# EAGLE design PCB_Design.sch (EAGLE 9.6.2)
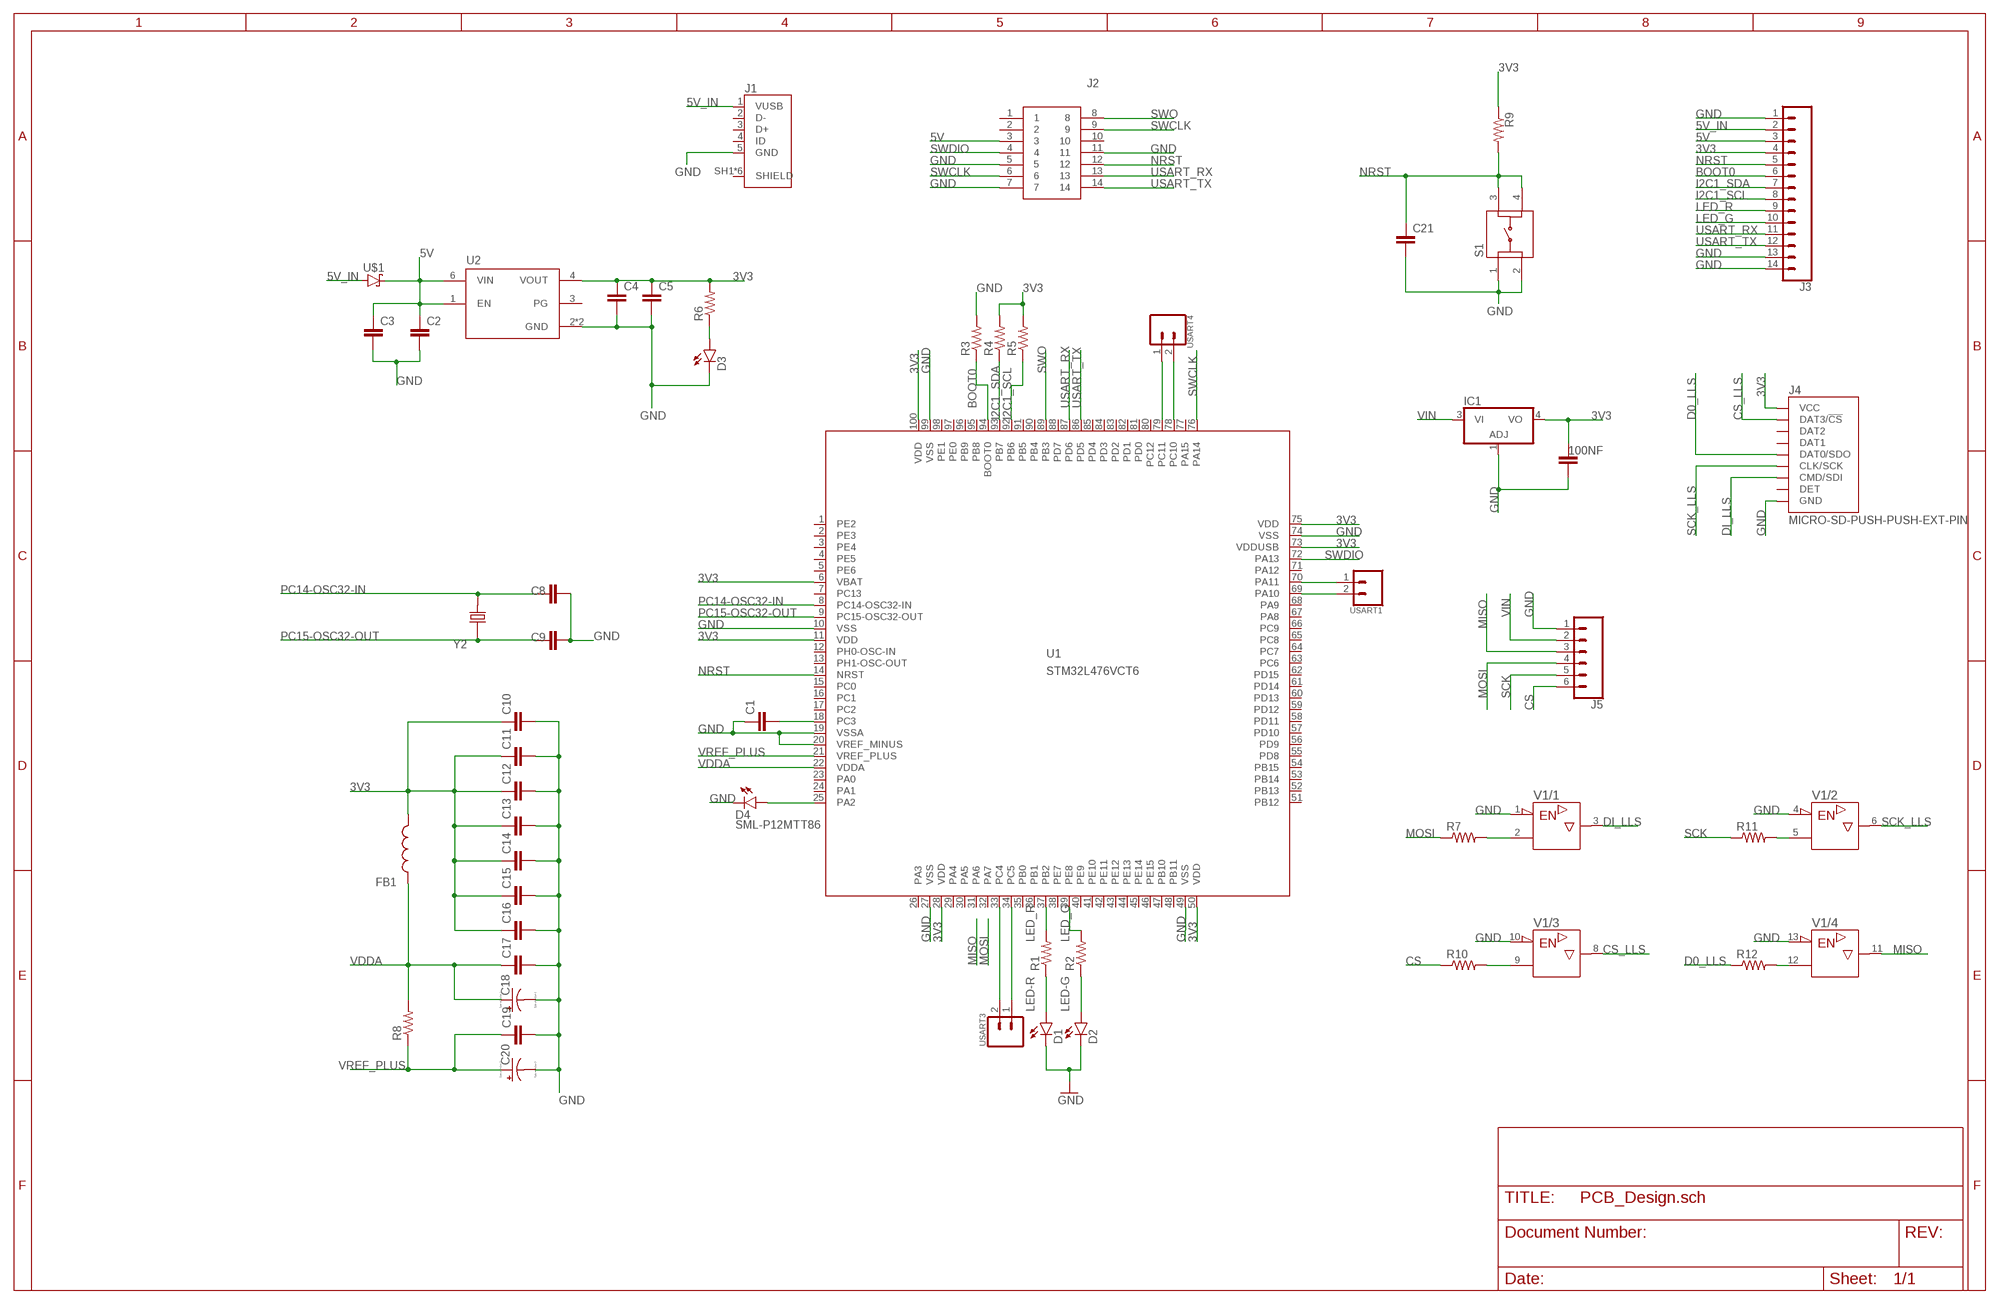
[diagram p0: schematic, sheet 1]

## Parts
100NF  C  (no package)
C1  CC0603KRX5R7BB105  [CAPC1608X90]
C2  CC0603KRX5R7BB105  [CAPC1608X90]
C3  CC0603KRX5R7BB105  [CAPC1608X90]
C4  CC0603KRX5R7BB105  [CAPC1608X90]
C5  CC0603KRX5R7BB105  [CAPC1608X90]
C8  CC0402CRNPO9BN4R7  [CAPC1005X55N]
C9  CC0402CRNPO9BN4R7  [CAPC1005X55N]
C10  CC0603KRX5R7BB105  [CAPC1608X90]
C11  CC0402KRX7R7BB104  [CAPC1005X55N]
C12  CC0402KRX7R7BB104  [CAPC1005X55N]
C13  CC0402KRX7R7BB104  [CAPC1005X55N]
C14  CC0402KRX7R7BB104  [CAPC1005X55N]
C15  CC0402KRX7R7BB104  [CAPC1005X55N]
C16  CC0402KRX7R7BB104  [CAPC1005X55N]
C17  CC0402KRX7R7BB104  [CAPC1005X55N]
C18  TAJA105K016RNJ  [CAPPM3216X180N]
C19  CC0402KRX7R7BB104  [CAPC1005X55N]
C20  TAJA105K016RNJ  [CAPPM3216X180N]
C21  CC0402KRX7R7BB104  [CAPC1005X55N]
D1  SML-P12MTT86  [LED_SML-P11UTT86R]
D2  SML-P12MTT86  [LED_SML-P11UTT86R]
D3  SML-P12VTT86  [LED_SML-P11UTT86R]
D4  SML-P12MTT86  [LED_SML-P11UTT86R]
FB1  BK1608HS601-T  [BEADC1608X95N]
IC1  317EMP  [SOT223]
J1  10118192-0001LF  [AMPHENOL_10118192-0001LF]
J2  FTSH-107-01-L-DV-K-A  [FTSH10701LDVKA]
J3  CONN_14  [1X14]
J4  MICRO-SD-PUSH-PUSH-EXT-PIN  [MICROSD-EXTERNALPIN]
J5  CONN_06LOCK  [1X06_LOCK]
R1  RC0402FR-071KL  [RESC1005X40N]
R2  RC0402FR-071KL  [RESC1005X40N]
R3  RC0402FR-071KL  [RESC1005X40N]
R4  RC0402FR-071KL  [RESC1005X40N]
R5  RC0402FR-071KL  [RESC1005X40N]
R6  RC0402FR-071KL  [RESC1005X40N]
R7  RC0402JR-070RL  [RESC1005X40]
R8  RC0402FR-071KL  [RESC1005X40N]
R9  RC0402FR-071KL  [RESC1005X40N]
R10  RC0402JR-070RL  [RESC1005X40]
R11  RC0402JR-070RL  [RESC1005X40]
R12  RC0402JR-070RL  [RESC1005X40]
S1  LL3301FF065QJ  [LL3301FF065QJ]
U1  STM32L476VCT6  [LQFP100_14X14]
U2  LD39050PU33R  [SON95P300X300X100-7N]
U$1  STPS1L30A  [DIOM5226X223N]
USART1  CONN_02LOCK  [1X02_LOCK]
USART3  CONN_02LOCK  [1X02_LOCK]
USART4  CONN_02LOCK  [1X02_LOCK]
V1  74125N  [DIL14]
Y2  ECS-.327-12.5-12QS-TR  [XTAL_ECS-.327-12.5-12QS-TR]

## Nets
3V3: 100NF.1 C4.1 C5.1 C10.1 C11.1 C12.1 C13.1 C14.1 C15.1 C16.1 FB1.2 IC1.4(VO) J3.4 J4.4(VCC) R4.2 R5.2 R6.2 R9.1 U1.6(VBAT) U1.11(VDD) U1.28(VDD) U1.50(VDD) U1.73(VDDUSB) U1.75(VDD) U1.100(VDD) U2.4(VOUT)
5V: C2.1 C3.1 J2.3 J3.3 U2.1(EN) U2.6(VIN) U$1.1(C)
5V_IN: J1.1(VUSB) J3.2 U$1.2(A)
BOOT0: J3.6 R3.1 U1.94(BOOT0)
CS: J5.6 R10.1
CS_LLS: J4.2(DAT3/!CS!) V1.8(/3:Y)
D0_LLS: J4.7(DAT0/SDO) R12.1
DI_LLS: J4.3(CMD/SDI) V1.3(/1:Y)
GND: 100NF.2 C1.1 C2.2 C3.2 C4.2 C5.2 C8.2 C9.2 C10.2 C11.2 C12.2 C13.2 C14.2 C15.2 C16.2 C17.2 C18.C(-) C19.2 C20.C(-) C21.2 D1.C D2.C D3.C D4.C IC1.1(ADJ) J1.5(GND) J2.5 J2.7 J2.11 J3.1 J3.13 J3.14 J4.6(GND) J4.10(GND) J4.11(GND) J4.12(GND) J4.13(GND) J5.1 R3.2 S1.1 S1.2 U1.10(VSS) U1.19(VSSA) U1.20(VREF_MINUS) U1.27(VSS) U1.49(VSS) U1.74(VSS) U1.99(VSS) U2.2(GND) U2.7(GND) V1.1(/1:!G) V1.4(/2:!G) V1.10(/3:!G) V1.13(/4:!G)
I2C1_SCL: J3.8 R5.1 U1.92(PB6)
I2C1_SDA: J3.7 R4.1 U1.93(PB7)
LED-G: D2.A R2.1
LED-R: D1.A R1.1
LED_G: J3.10 R2.2 U1.39(PE8)
LED_R: J3.9 R1.2 U1.37(PB2)
MISO: J5.3 V1.11(/4:Y)
MOSI: J5.4 R7.1
N$1: D4.A U1.25(PA2)
N$2: U1.33(PC4) USART3.2
N$3: U1.34(PC5) USART3.1
N$4: U1.78(PC10) USART4.2
N$5: U1.69(PA10) USART1.2
N$6: U1.79(PC11) USART4.1
N$7: U1.70(PA11) USART1.1
N$9: R7.2 V1.2(/1:A)
N$10: R10.2 V1.9(/3:A)
N$11: C1.2 U1.18(PC3)
N$13: R11.2 V1.5(/2:A)
N$14: D3.A R6.1
N$17: R12.2 V1.12(/4:A)
NRST: C21.1 J2.12 J3.5 R9.2 S1.3 S1.4 U1.14(NRST)
PC14-OSC32-IN: C8.1 U1.8(PC14-OSC32-IN) Y2.2
PC15-OSC32-OUT: C9.1 U1.9(PC15-OSC32-OUT) Y2.1
SCK: J5.5 R11.1
SCK_LLS: J4.5(CLK/SCK) V1.6(/2:Y)
SWCLK: J2.6 J2.9 U1.76(PA14)
SWDIO: J2.4 U1.72(PA13)
SWO: J2.8 U1.89(PB3)
USART_RX: J2.13 J3.11 U1.87(PD6)
USART_TX: J2.14 J3.12 U1.86(PD5)
VDDA: C17.1 C18.A(+) FB1.1 R8.2 U1.22(VDDA)
VIN: IC1.3(VI) J5.2
VREF_PLUS: C19.1 C20.A(+) R8.1 U1.21(VREF_PLUS)
Unconnected: J1.2(D-) J1.3(D+) J1.4(ID) J1.SH1(SHIELD) J1.SH2(SHIELD) J1.SH3(SHIELD) J1.SH4(SHIELD) J1.SH5(SHIELD) J1.SH6(SHIELD) J2.1 J2.2 J2.10 J4.1(DAT2) J4.8(DAT1) J4.9(DET) U1.1(PE2) U1.2(PE3) U1.3(PE4) U1.4(PE5) U1.5(PE6) U1.7(PC13) U1.12(PH0-OSC-IN) U1.13(PH1-OSC-OUT) U1.15(PC0) U1.16(PC1) U1.17(PC2) U1.23(PA0) U1.24(PA1) U1.26(PA3) U1.29(PA4) U1.30(PA5) U1.31(PA6) U1.32(PA7) U1.35(PB0) U1.36(PB1) U1.38(PE7) U1.40(PE9) U1.41(PE10) U1.42(PE11) U1.43(PE12) U1.44(PE13) U1.45(PE14) U1.46(PE15) U1.47(PB10) U1.48(PB11) U1.51(PB12) U1.52(PB13) U1.53(PB14) U1.54(PB15) U1.55(PD8) U1.56(PD9) U1.57(PD10) U1.58(PD11) U1.59(PD12) U1.60(PD13) U1.61(PD14) U1.62(PD15) U1.63(PC6) U1.64(PC7) U1.65(PC8) U1.66(PC9) U1.67(PA8) U1.68(PA9) U1.71(PA12) U1.77(PA15) U1.80(PC12) U1.81(PD0) U1.82(PD1) U1.83(PD2) U1.84(PD3) U1.85(PD4) U1.88(PD7) U1.90(PB4) U1.91(PB5) U1.95(PB8) U1.96(PB9) U1.97(PE0) U1.98(PE1) U2.3(PG)

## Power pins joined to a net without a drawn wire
+UB: V1.14(/+UB:+UB)
-UB: V1.7(/-UB:-UB)

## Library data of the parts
100NF = ngspice-simulation:C: CAPACITOR
C1-C5 C10 = ce-capstone:CC0603KRX5R7BB105: CAPACITOR CERAMIC, 1µF, 10V, X5R, 0603; Dielectric Characteristic:X5R; Capacitance:1µF; Capacitance Tolerance:± 10%; Voltage Rating:16V; Temperature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; DESCRIPTION: 1µF ±10% 16V Ceramic Capacitor X5R 0603 _1608 Metric_; DIGI-KEY_PART_NUMBER: 311-1444-1-ND; DIGI-KEY_PURCHASE_URL: https://www.digikey.com/product-detail/en/yageo/CC0603KRX5R7BB105/311-1444-1-ND/2833750?utm_source=snapeda&utm_medium=aggregator&utm_campaign=symbol; MF: Yageo; MP: CC0603KRX5R7BB105; PACKAGE: 0603 Yageo
C8 C9 = ce-capstone:CC0402CRNPO9BN4R7: 0402 4.7 pF 50 V ±0.25 pF Tolerance NP0 SMT Multilayer Ceramic Capacitor; DESCRIPTION: 4.7pF ±0.25pF 50V Ceramic Capacitor C0G, NP0 0402 _1005 Metric_; DIGI-KEY_PART_NUMBER: 311-1367-1-ND; DIGI-KEY_PURCHASE_URL: https://www.digikey.com/product-detail/en/yageo/CC0402CRNPO9BN4R7/311-1367-1-ND/2103151?utm_source=snapeda&utm_medium=aggregator&utm_campaign=symbol; MF: Yageo; MP: CC0402CRNPO9BN4R7; PACKAGE: 0402 Yageo
C11-C17 C19 C21 = ce-capstone:CC0402KRX7R7BB104: .1UF 16V 10% 0402; DESCRIPTION: 0.1µF ±10% 16V Ceramic Capacitor X7R 0402 _1005 Metric_; DIGI-KEY_PART_NUMBER: 311-1338-1-ND; DIGI-KEY_PURCHASE_URL: https://www.digikey.com/product-detail/en/yageo/CC0402KRX7R7BB104/311-1338-1-ND/2103122?utm_source=snapeda&utm_medium=aggregator&utm_campaign=symbol; MF: Yageo; MP: CC0402KRX7R7BB104; PACKAGE: 0402 Yageo
C18 C20 = ce-capstone:TAJA105K016RNJ: Capacitor tantalum TAJ 1206 1uF 16V AVX 1uF SMD Solid MnO2 Tantalum Electrolytic Capacitor, 16 V dc +/-10%, TAJ Series; ALLIED_NUMBER: 70474975; ALLIED_PRICE-STOCK: https://www.alliedelec.com/avx-taja105k016r/70474975/; DESCRIPTION: Capacitor tantalum TAJ 1206 1uF 16V AVX 1uF SMD Solid MnO2 Tantalum Electrolytic Capacitor, 16 V dc +/-10%, TAJ Series; HEIGHT: 1.8mm; MANUFACTURER_NAME: AVX; MANUFACTURER_PART_NUMBER: TAJA105K016RNJ; MOUSER_PART_NUMBER: 581-TAJA105K016RNJ; MOUSER_PRICE-STOCK: https://www.mouser.com/Search/Refine.aspx?Keyword=581-TAJA105K016R; RS_PART_NUMBER: 6992804P; RS_PRICE-STOCK: http://uk.rs-online.com/web/p/products/6992804P
D1 D2 D4 = ce-capstone:SML-P12MTT86: SML-P1 Series Red 0402 Clear 60 mcd 2 V Surface Mount PICOLED LED; AVAILABILITY: Unavailable; DESCRIPTION: Green 572nm LED Indication - Discrete 2V 0402 _1006 Metric_; MF: Rohm; MP: SML-P12MTT86; PACKAGE: 0402 Rohm; PRICE: None
D3 = ce-capstone:SML-P12VTT86: SML-P1 Series Red 0402 Clear 60 mcd 2 V Surface Mount PICOLED LED; AVAILABILITY: Unavailable; DESCRIPTION: Red 630nm LED Indication - Discrete 2V 0402 _1006 Metric_; MF: Rohm; MP: SML-P12VTT86; PACKAGE: 0402 Rohm; PRICE: None
FB1 = ce-capstone:BK1608HS601-T: Ferrite Chip Bead(Lead Free); DESCRIPTION: Ferrite Chip Bead(Lead Free); HEIGHT: 0.95mm; MANUFACTURER_NAME: Taiyo Yuden; MANUFACTURER_PART_NUMBER: BK1608HS601-T
IC1 = linear:*317: Positive VOLTAGE REGULATOR
J1 = ce-capstone:10118192-0001LF: Single Port 5 Contact Horizontal Right Angle Shielded Micro B USB 2.0 Connector; AVAILABILITY: Unavailable; DESCRIPTION: USB - micro B USB 2.0 Receptacle Connector 5 Position Surface Mount, Right Angle; MF: Amphenol ICC; MP: 10118192-0001LF; PACKAGE: None; PRICE: None
J2 = ce-capstone:FTSH-107-01-L-DV-K-A: Headers & Wire Housings .050" Micro Terminal Strip Source: Datasheet; DESCRIPTION: Headers & Wire Housings .050" Micro Terminal Strip; HEIGHT: 5.97mm; MANUFACTURER_NAME: SAMTEC; MANUFACTURER_PART_NUMBER: FTSH-107-01-L-DV-K-A; MOUSER_PART_NUMBER: 200-FTSH10701LDVKA; MOUSER_PRICE-STOCK: https://www.mouser.com/Search/Refine.aspx?Keyword=200-FTSH10701LDVKA
J3 = SparkFun-Connectors:CONN_14: Multi connection point. Often used as Generic Header-pin footprint for 0.1 inch spaced/style header connections On any of the 0.1 inch spaced packages, you can populate with these: Break Away Headers - Straight (PRT-00116) Break Away Male Headers - Right Angle (PRT-00553) Female Headers (PRT-00115)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
J4 = SparkFun-Connectors:MICRO-SD: microSD Socket for Transflash Various sockets for µSD. tDoc lines correctly indicate media card edge positions when inserting (unlocked, locked, depressed). NOTE: CD1 and CD2 are connected internally, and the default detect state of the socket is detect pin to ground. SparkFun Products: WAV Trigger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; PROD_ID: CONN-16110
J5 = SparkFun-Connectors:CONN_06: Multi connection point. Often used as Generic Header-pin footprint for 0.1 inch spaced/style header connections On any of the 0.1 inch spaced packages, you can populate with these: Break Away Headers - Straight (PRT-00116) Break Away Male Headers - Right Angle (PRT-00553) Female Headers (PRT-00115)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
R1-R6 R8 R9 = ce-capstone:RC0402FR-071KL: RES SMD 1k OHM 1% 1/16W 0402; DESCRIPTION: 510 Ohms ±1% 0.063W, 1/16W Chip Resistor 0402 _1005 Metric_ Moisture Resistant Thick Film; DIGI-KEY_PART_NUMBER: 311-510LRCT-ND; DIGI-KEY_PURCHASE_URL: https://www.digikey.com/product-detail/en/yageo/RC0402FR-07510RL/311-510LRCT-ND/729579?utm_source=snapeda&utm_medium=aggregator&utm_campaign=symbol; MF: Yageo; MP: RC0402FR-07510RL; PACKAGE: 1005 Panasonic Electronic Components
R7 R10-R12 = ce-capstone:RC0402JR-070RL: RC Series 0402 62.5 mW 0 Ohms 5% ±200 ppm/°C SMT Thick Film Chip Resistor; AVAILABILITY: Unavailable; DESCRIPTION: 0 Ohms Jumper 0.063W, 1/16W Chip Resistor 0402 _1005 Metric_ Moisture Resistant Thick Film; MF: Yageo; MP: RC0402JR-070RL; PACKAGE: 0402 Yageo; PRICE: None
S1 = ce-capstone:LL3301FF065QJ: Pushbutton Switches 50mA 12VDC F065 7.0mm J-Lead Source: Datasheet; DESCRIPTION: Pushbutton Switches 50mA 12VDC F065 7.0mm J-Lead; HEIGHT: 7.3mm; MANUFACTURER_NAME: E-Switch; MANUFACTURER_PART_NUMBER: LL3301FF065QJ; MOUSER_PART_NUMBER: 612-LL3301FF065QJ; MOUSER_PRICE-STOCK: https://www.mouser.com/Search/Refine.aspx?Keyword=612-LL3301FF065QJ
U1 = ce-capstone:STM32L476V*: STM32L476VX LQFP100 Datasheet STM32L476XX; FARNELL: 2518171; FLASH: 256kB; SRAM: 128kB
U2 = ce-capstone:LD39050PU33R: LD39050 Series 500 mA 3.3 V Fixed Low Noise LDO Voltage Regulator - DFN-6; AVAILABILITY: Unavailable; DESCRIPTION: Linear Voltage Regulator IC 1 Output 500mA 6-DFN _3x3_; MF: STMicroelectronics; MP: LD39050PU33R; PACKAGE: DFN-6 STMicroelectronics; PRICE: None
U$1 = ce-capstone:STPS1L30A
USART1 USART3 USART4 = SparkFun-Connectors:CONN_02: Multi connection point. Often used as Generic Header-pin footprint for 0.1 inch spaced/style header connections
V1 = 74ttl-din:74*125: Quad bus BUFFER, 3-state
Y2 = ce-capstone:ECS-.327-12.5-12QS-TR: SMD CRYSTAL 32.768 KHz; AVAILABILITY: Unavailable; DESCRIPTION: 32.768kHz ±20ppm Crystal 12.5pF 90 kOhms 2-SMD, No Lead; MF: ECS Inc.; MP: ECS-.327-12.5-12QS-TR; PACKAGE: SMD-2 ECS International; PRICE: None

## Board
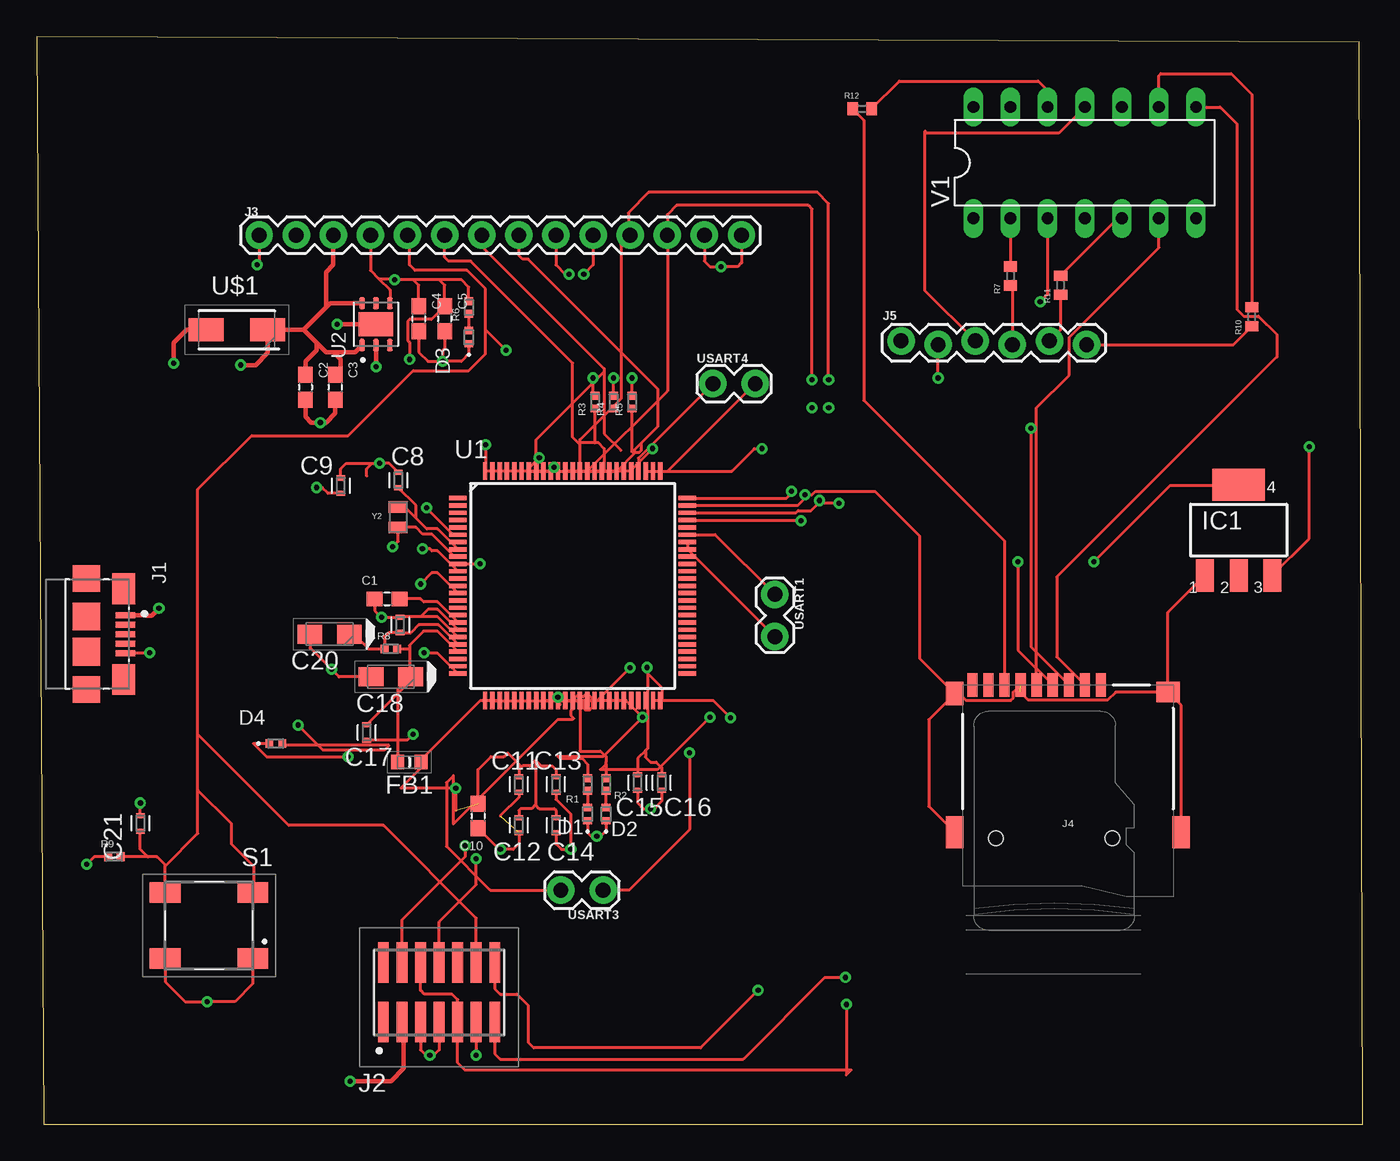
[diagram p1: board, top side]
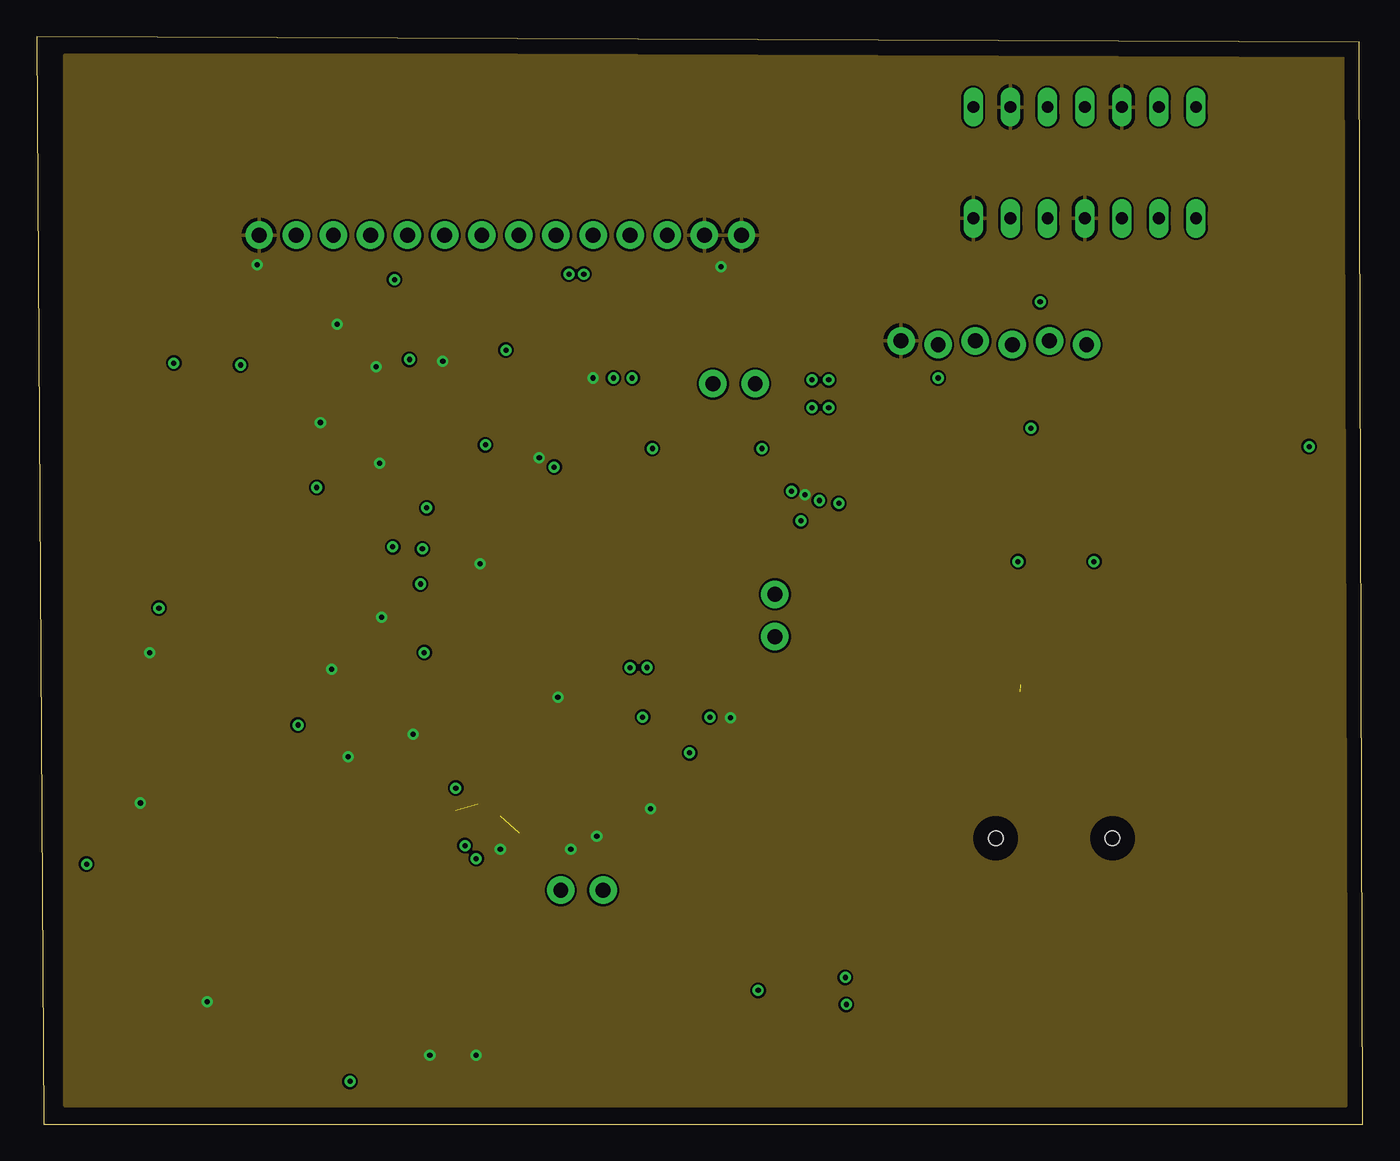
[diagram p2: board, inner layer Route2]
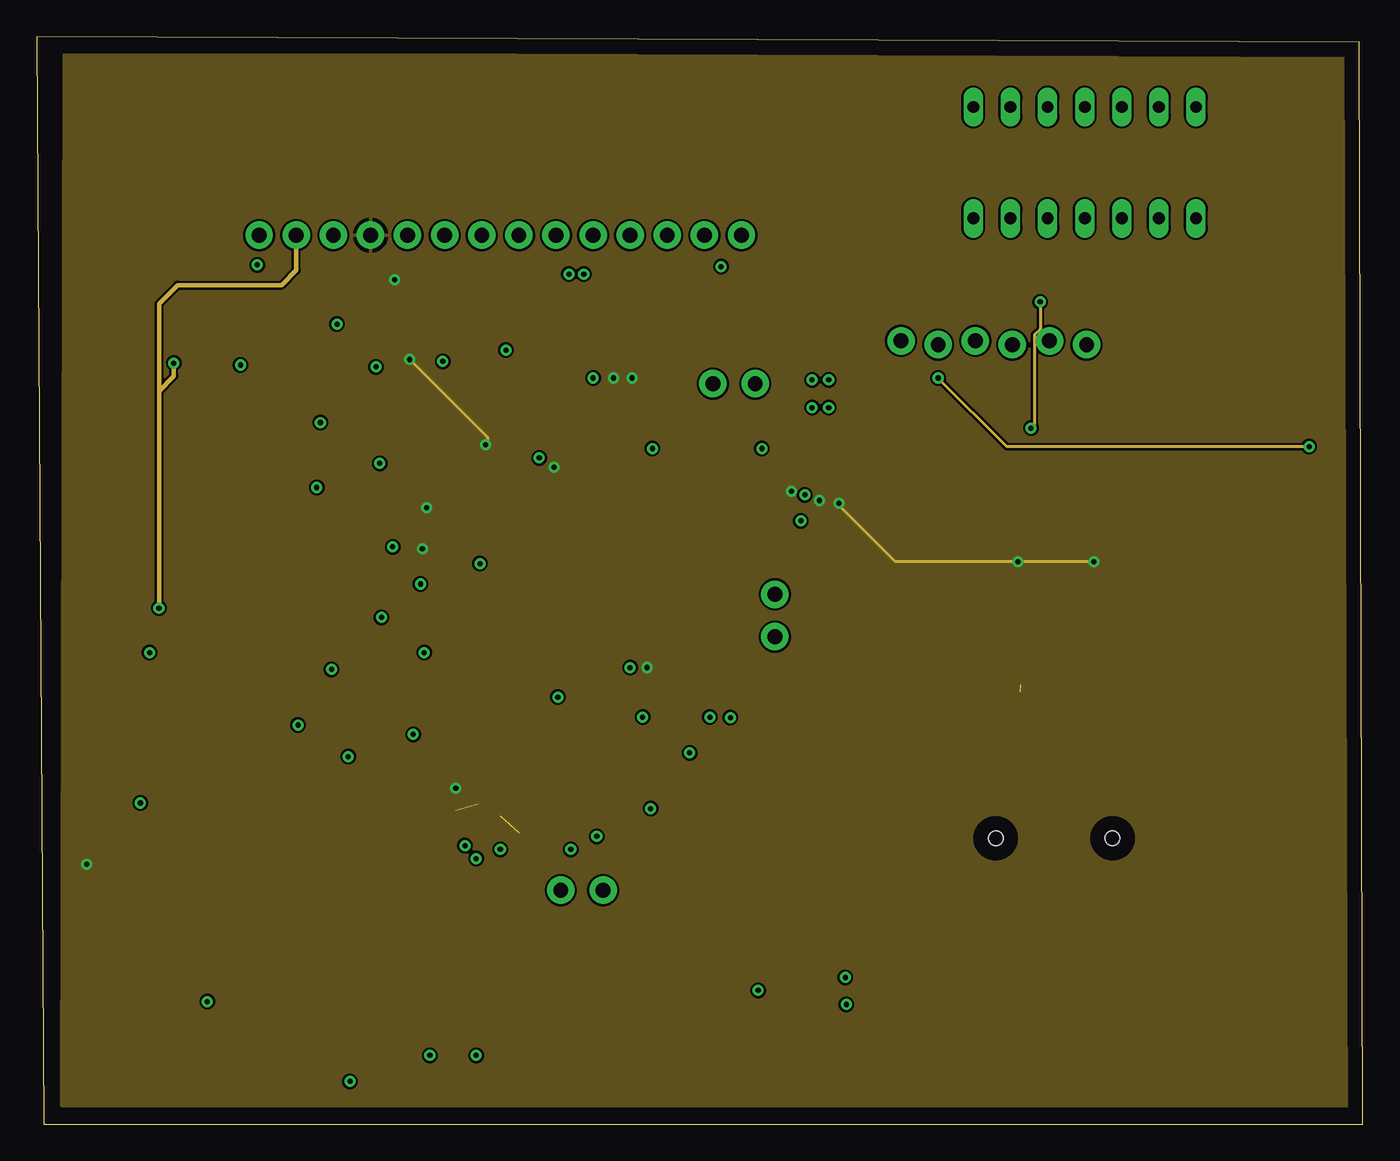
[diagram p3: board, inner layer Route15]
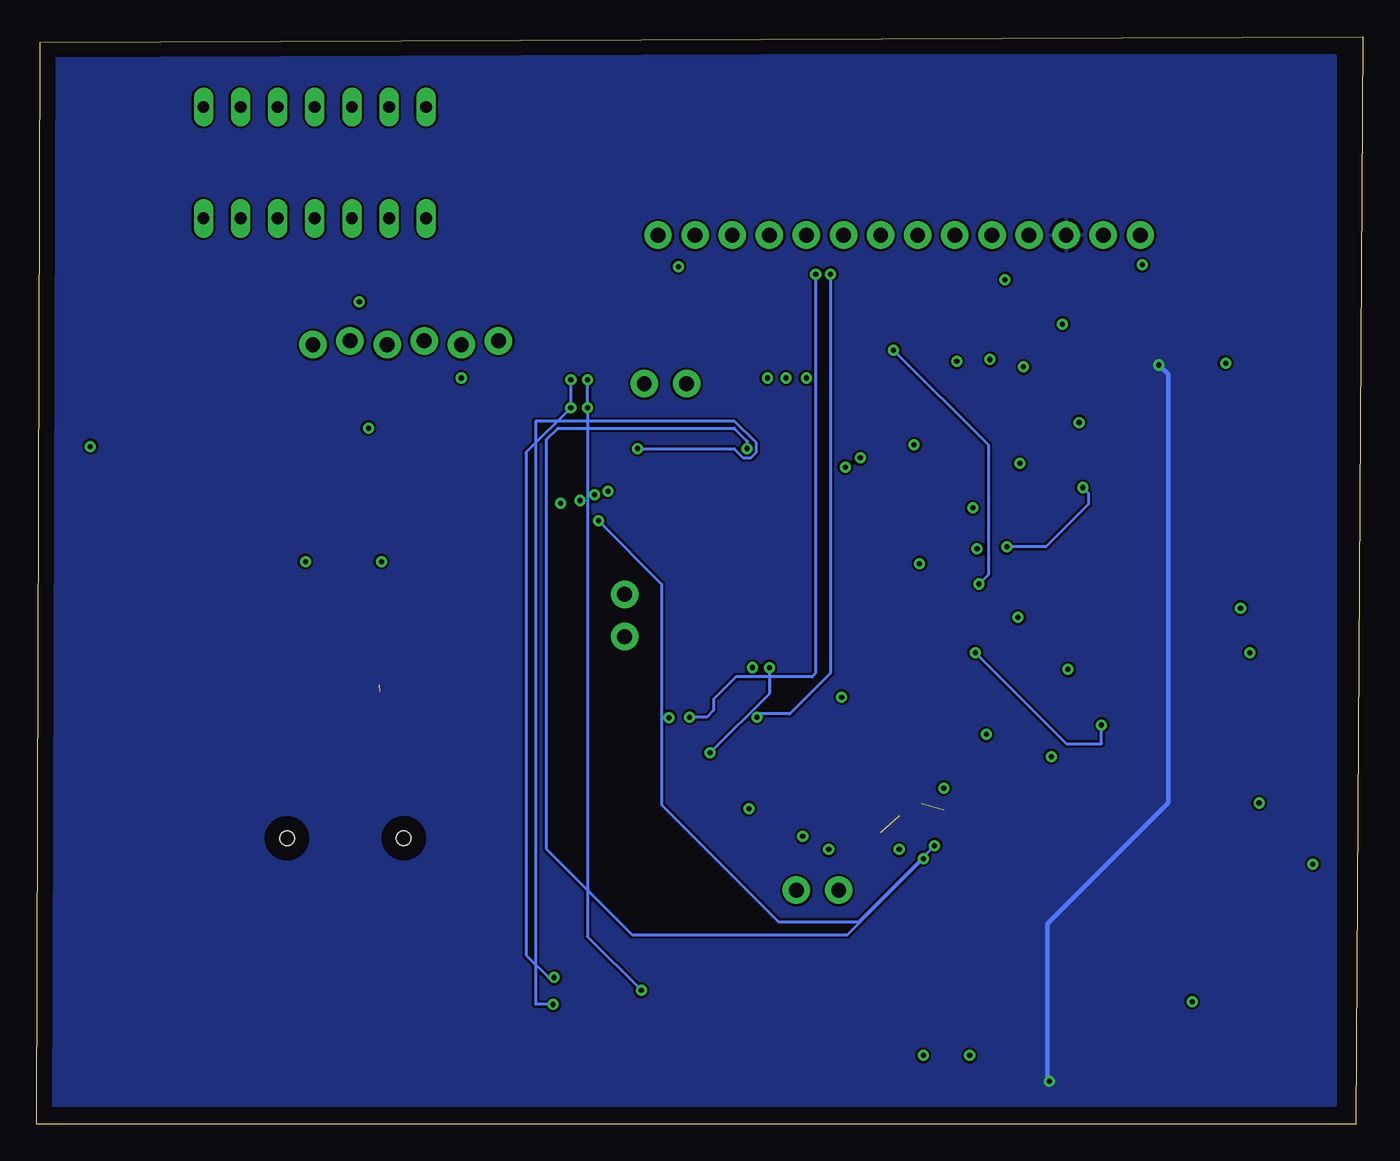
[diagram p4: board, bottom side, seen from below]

Size 90.81 x 74.42 mm. Coordinates in mm from the lower left corner, seen from the top.
Outline: 0.51,0 90.81,0 90.55,74.04 0,74.42 0.51,0
Copper layers (1+2*15+16): Top 0.035mm / dielectric 1.5mm / Route2 0.035mm / dielectric 0.15mm / Route15 0.035mm / dielectric 0.2mm / Bottom 0.035mm
Design rules "default *": minimum track width 8mil, minimum drill 0.35mm, track to track 6mil, track to pad 6mil, pad to pad 6mil, via to via 6mil, smd to smd 6mil, copper to edge 40mil, drill to drill 6mil, minimum pad ring 10mil, minimum via ring 8mil, stop-mask expansion 4mil, vias tented up to drill 0mil, thermal gap 10mil

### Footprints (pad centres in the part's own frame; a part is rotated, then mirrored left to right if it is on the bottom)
CAPC1608X90 = smd 1.1 x 1: 1 -0.85,0; 2 0.85,0
CAPC1005X55N = smd 0.35 x 0.6: 1 -0.525,0; 2 0.525,0
CAPPM3216X180N = smd 1.7 x 1.3: A -1.35,0; C 1.35,0
LED_SML-P11UTT86R = smd 0.5 x 0.6: A 0.45,0; C -0.45,0
BEADC1608X95N = smd 0.9 x 1: 1 -0.8,0; 2 0.8,0
SOT223 = smd 1.219 x 2.235: 1 -2.311,-3.099; 2 0,-3.099; 3 2.311,-3.099 | smd 3.6 x 2.2: 4 0,3.099
AMPHENOL_10118192-0001LF = smd 0.4 x 1.35: 1 -1.3,0; 2 -0.65,0; 3 0,0; 4 0.65,0; 5 1.3,0 | smd 2.1 x 1.6: SH1 -3.1,-0.125; SH2 3.1,-0.125 | smd 1.8 x 1.9: SH3 -3.8,-2.675; SH6 3.8,-2.675 | smd 1.9 x 1.9: SH4 -1.2,-2.675; SH5 1.2,-2.675
FTSH10701LDVKA = smd 0.74 x 2.79: 1 -3.81,-2.035; 2 -3.81,2.035; 3 -2.54,-2.035; 4 -2.54,2.035; 5 -1.27,-2.035; 6 -1.27,2.035; 7 0,-2.035; 8 0,2.035; 9 1.27,-2.035; 10 1.27,2.035; 11 2.54,-2.035; 12 2.54,2.035; 13 3.81,-2.035; 14 3.81,2.035
1X14 = drill 1.016 pad 1.88: 1 0,0; 2 2.54,0; 3 5.08,0; 4 7.62,0; 5 10.16,0; 6 12.7,0; 7 15.24,0; 8 17.78,0; 9 20.32,0; 10 22.86,0; 11 25.4,0; 12 27.94,0; 13 30.48,0; 14 33.02,0
MICROSD-EXTERNALPIN = smd 0.7 x 1.6: 1 2.25,10.5; 2 1.15,10.5; 3 0.05,10.5; 4 -1.05,10.5; 5 -2.15,10.5; 6 -3.25,10.5; 7 -4.35,10.5; 8 -5.45,10.5; 9 -6.55,10.5 | smd 1.2 x 1.6: 10 -7.75,9.9 | smd 1.2 x 2.2: 11 -7.75,0.4; 12 7.75,0.4 | smd 1.6 x 1.4: 13 6.85,10 | hole 1: 3.05,0; -4.95,0
1X06_LOCK = drill 1.016 pad 1.88: 1 0,0; 2 2.54,-0.254; 3 5.08,0; 4 7.62,-0.254; 5 10.16,0; 6 12.7,-0.254
RESC1005X40N = smd 0.54 x 0.6: 1 -0.432,0; 2 0.432,0
RESC1005X40 = smd 0.7 x 0.9: 1 -0.65,0; 2 0.65,0
LL3301FF065QJ = smd 2.1 x 1.4: 1 -3,2.25; 2 3,2.25; 3 -3,-2.25; 4 3,-2.25
LQFP100_14X14 = smd 1.2 x 0.3: 1 -7.85,6; 2 -7.85,5.5; 3 -7.85,5; 4 -7.85,4.5; 5 -7.85,4; 6 -7.85,3.5; 7 -7.85,3; 8 -7.85,2.5; 9 -7.85,2; 10 -7.85,1.5; 11 -7.85,1; 12 -7.85,0.5; 13 -7.85,0; 14 -7.85,-0.5; 15 -7.85,-1; 16 -7.85,-1.5; 17 -7.85,-2; 18 -7.85,-2.5; 19 -7.85,-3; 20 -7.85,-3.5; 21 -7.85,-4; 22 -7.85,-4.5; 23 -7.85,-5; 24 -7.85,-5.5; 25 -7.85,-6; 51 7.85,-6; 52 7.85,-5.5; 53 7.85,-5; 54 7.85,-4.5; 55 7.85,-4; 56 7.85,-3.5; 57 7.85,-3; 58 7.85,-2.5; 59 7.85,-2; 60 7.85,-1.5; 61 7.85,-1; 62 7.85,-0.5; 63 7.85,0; 64 7.85,0.5; 65 7.85,1; 66 7.85,1.5; 67 7.85,2; 68 7.85,2.5; 69 7.85,3; 70 7.85,3.5; 71 7.85,4; 72 7.85,4.5; 73 7.85,5; 74 7.85,5.5; 75 7.85,6 | smd 0.3 x 1.2: 26 -6,-7.85; 27 -5.5,-7.85; 28 -5,-7.85; 29 -4.5,-7.85; 30 -4,-7.85; 31 -3.5,-7.85; 32 -3,-7.85; 33 -2.5,-7.85; 34 -2,-7.85; 35 -1.5,-7.85; 36 -1,-7.85; 37 -0.5,-7.85; 38 0,-7.85; 39 0.5,-7.85; 40 1,-7.85; 41 1.5,-7.85; 42 2,-7.85; 43 2.5,-7.85; 44 3,-7.85; 45 3.5,-7.85; 46 4,-7.85; 47 4.5,-7.85; 48 5,-7.85; 49 5.5,-7.85; 50 6,-7.85; 76 6,7.85; 77 5.5,7.85; 78 5,7.85; 79 4.5,7.85; 80 4,7.85; 81 3.5,7.85; 82 3,7.85; 83 2.5,7.85; 84 2,7.85; 85 1.5,7.85; 86 1,7.85; 87 0.5,7.85; 88 0,7.85; 89 -0.5,7.85; 90 -1,7.85; 91 -1.5,7.85; 92 -2,7.85; 93 -2.5,7.85; 94 -3,7.85; 95 -3.5,7.85; 96 -4,7.85; 97 -4.5,7.85; 98 -5,7.85; 99 -5.5,7.85; 100 -6,7.85
SON95P300X300X100-7N = smd 0.84 x 0.4: 1 -1.435,0.95; 2 -1.435,0; 3 -1.435,-0.95; 4 1.435,-0.95; 5 1.435,0; 6 1.435,0.95 | smd 1.625 x 2.365: 7 0,0
DIOM5226X223N = smd 2.4 x 1.55: 1 -2.1,0; 2 2.1,0
1X02_LOCK = drill 1.016 pad 1.88: 1 -0.178,0; 2 2.718,0
DIL14 = drill 0.813 long: 1 -7.62,-3.81; 2 -5.08,-3.81; 3 -2.54,-3.81; 4 0,-3.81; 5 2.54,-3.81; 6 5.08,-3.81; 7 7.62,-3.81; 8 7.62,3.81; 9 5.08,3.81; 10 2.54,3.81; 11 0,3.81; 12 -2.54,3.81; 13 -5.08,3.81; 14 -7.62,3.81
XTAL_ECS-.327-12.5-12QS-TR = smd 0.8 x 1.3: 1 -0.7,0; 2 0.7,0

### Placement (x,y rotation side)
C1  24,35.94 0 top
C2  18.42,50.42 270 top
C3  20.45,50.42 270 top
C4  26.16,55.12 270 top
C5  27.94,55.12 270 top
C8  24.77,44.07 90 top
C9  20.83,43.69 90 top
C10  30.23,21.08 270 top
C11  33.02,23.24 270 top
C12  33.02,20.45 270 top
C13  35.56,23.24 270 top
C14  35.56,20.45 270 top
C15  41.15,23.37 270 top
C16  42.8,23.37 270 top
C17  22.61,26.8 270 top
C18  24.26,30.61 180 top
C19  24.89,34.16 90 top
C20  20.07,33.53 180 top
C21  7.11,20.57 90 top
D1  37.72,21.21 90 top
D2  38.99,21.21 90 top
D3  29.59,53.85 90 top
D4  16.38,26.04 0 top
FB1  25.53,24.77 0 top
IC1  82.3,40.64 0 top
J1  6.1,33.53 270 top
J2  27.56,9.02 0 top
J3  15.24,60.83 0 top
J4  70.61,19.56 0 top
J5  59.18,53.59 0 top
R1  37.72,23.24 90 top
R2  38.99,23.24 90 top
R3  38.23,49.4 90 top
R4  39.5,49.4 90 top
R5  40.77,49.4 90 top
R6  29.59,55.88 90 top
R7  66.68,58.04 90 top
R8  24.26,32.51 0 top
R9  5.33,18.29 0 top
R10  83.19,55.24 90 top
R11  70.1,57.4 90 top
R12  56.52,69.47 0 top
S1  11.81,13.59 180 top
U1  36.7,36.83 0 top
U2  23.24,54.74 90 top
U$1  13.72,54.36 180 top
USART1  50.55,36.07 270 top
USART3  38.61,16 180 top
USART4  46.48,50.67 0 top
V1  71.76,65.79 0 top
Y2  24.77,41.53 90 top

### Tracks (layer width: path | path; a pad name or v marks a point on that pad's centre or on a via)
3V3  (via drill 0.35)  (1 unrouted)
  Top 0.203: U1.28 30.38,28.98 26.33,24.93 FB1.2 26.33,24.38 24.93,22.99 v28.7,22.99 28.7,21.46 | U1.50 42.83,29.11 42.83,29.84 41.81,30.86 | 41.81,30.86 41.81,25.68 41.69,25.56 | 41.69,25.56 41.15,25.02 C15.1 | 41.69,25.56 41.69,25.11 42.04,24.77 42.42,24.77 42.8,24.38 C16.1 | 34.16,24.89 33.78,24.51 33.27,24.51 33.02,24.26 C11.1 33.02,24.64 32.26,25.4 32,25.15 31.12,25.15 30.23,24.26 C10.1 | 34.16,24.89 34.54,24.51 35.31,24.51 35.56,24.26 C13.1 | 34.16,24.89 34.16,21.84 | 34.16,21.84 33.91,21.59 33.15,21.59 33.02,21.46 C12.1 | 34.16,21.84 34.42,21.59 35.43,21.59 35.56,21.46 C14.1 | R4.2 v39.5,51.05 | R5.2 v40.77,51.05 | v41.78,31.24 41.78,30.89 41.81,30.86 | J3.4 22.86,58.42 23.43,57.85 | U2.4 24.19,57.09 23.43,57.85 | 23.43,57.85 24.45,57.85 v24.51,57.78 25.78,57.78 | C4.1 26.16,57.4 25.78,57.78 | 27.56,57.78 27.94,57.4 C5.1 27.04,55.07 25.56,55.07 25.41,54.92 25.41,53.61 25.53,53.49 v25.53,52.32 | 27.56,57.78 25.78,57.78 | R6.2 29.59,57.28 29.08,57.78 27.56,57.78 | R9.1 3.94,18.29 v3.43,17.78 | U1.75 51.34,42.83 51.69,43.18 v51.69,43.31 | U1.73 51.98,41.83 52.13,41.97 53.02,41.97 53.59,42.55 v53.59,42.67 53.78,42.48 v54.93,42.48 | U1.6 28.5,40.33 26.71,42.13 v26.71,42.16 | U1.11 27.46,39.23 27.07,39.23 26.94,39.36 v26.42,39.36 | v35.43,44.96 35.16,44.68 30.8,44.68 | 30.8,44.68 U1.100 | IC1.4 82.25,43.69 77.6,43.69 v72.39,38.48 | v67.18,38.48 67.18,32.44 J4.4 | v30.73,46.48 30.73,44.81 30.8,44.74 30.8,44.68
  Route15 0.203: v72.39,38.48 v67.18,38.48 58.8,38.48 54.86,42.42 v54.93,42.48 | v25.53,52.32 30.86,46.99 30.86,46.61 v30.73,46.48
  pour Route15: 1.7,1.27 89.79,1.27 89.79,73.15 1.86,73.15
5V  (via drill 0.35)
  Top 0.305: 18.29,54.36 U$1.1 15.82,52.77 14.99,51.94 v13.97,51.94 | J3.3 20.32,58.8 19.81,58.29 19.81,55.88 | 18.29,54.36 19.81,55.88 | 19.81,55.88 20.1,56.17 U2.6 | 18.29,54.36 19.18,53.47 | 19.18,53.47 19.18,52.96 18.42,52.2 C2.1 | 19.18,53.47 19.81,52.83 20.32,52.83 | U2.1 21.82,52.83 20.32,52.83 | 20.32,52.83 20.83,52.32 20.83,51.65 C3.1 | v21.46,2.92 24.26,2.92 25.15,3.81 25.15,6.86 J2.3
  Bottom 0.305: v13.97,51.94 13.33,51.31 13.33,21.97 21.59,13.72 21.59,3.05 v21.46,2.92
  pour Bottom: 1.91,73.15 1.91,1.27 89.79,1.27 89.79,73.15
5V_IN  (via drill 0.35)
  Top 0.305: J1.1 7.46,34.83 7.49,34.8 7.87,34.8 v8.38,35.31 | v9.4,52.07 9.4,53.47 10.29,54.36 U$1.2
  Route15 0.305: v8.38,35.31 8.38,50.16 | 8.38,50.16 8.38,53.21 8.38,56.13 9.65,57.4 16.76,57.4 17.78,58.42 J3.2 | 8.38,50.16 9.4,51.18 v9.4,52.07
BOOT0
  Top 0.203: U1.94 38.86,44.68 38.86,46.23 38.48,46.61 38.23,46.61 | 38.23,46.61 R3.1 | 38.23,46.61 37.08,46.61 36.7,46.99 36.7,52.07 29.72,59.05 28.19,59.05 27.94,59.31 J3.6
CS
  Top 0.203: J5.6 81.93,53.34 R10.1
CS_LLS
  Top 0.203: V1.8 81.03,69.6 82.17,68.45 82.17,55.75 82.63,55.29 83.65,55.29 84.91,54.03 84.91,52.5 69.84,37.44 69.84,31.98 J4.2
D0_LLS
  Top 0.203: R12.1 56.64,68.69 56.64,49.53 66.26,39.91 J4.7
DI_LLS  (via drill 0.35)
  Top 0.203: V1.3 69.22,56.77 v68.71,56.26 | v68.07,47.62 68.07,32.65 J4.3
  Route15 0.203: v68.71,56.26 68.71,54.4 68.33,54.02 68.33,47.88 v68.07,47.62
GND  (via drill 0.35)  (2 unrouted)
  Top 0.203: J1.5 6.13,32.26 v7.75,32.26 | U1.20 27.46,34.73 26.29,34.73 | 26.29,34.73 24.93,34.73 C19.2 24.89,34.67 v23.62,34.67 23.15,35.14 C1.1 | U1.19 27.46,35.23 26.79,35.23 26.29,34.73 | C20.C 18.72,32.59 v20.19,31.11 20.7,30.61 C18.C | v25.78,26.67 25.38,26.27 C17.2 | C13.2 35.56,22.23 36.58,21.21 v36.58,18.8 35.94,18.8 35.56,19.18 C14.2 | C11.2 33.02,22.35 31.75,21.08 | C15.2 41.15,21.97 41.53,21.59 v42.04,21.59 42.29,21.59 42.8,22.1 C16.2 | v47.5,27.81 46.33,28.98 U1.49 | C10.2 31.66,18.8 v31.75,18.8 32.64,18.8 33.02,19.18 C12.2 | D1.C 37.72,19.94 37.97,19.69 v38.35,19.69 38.61,19.69 38.99,20.07 D2.C | C8.2 24.15,45.21 v23.5,45.21 22.99,45.21 | 22.61,44.34 22.61,44.83 22.99,45.21 | C9.2 20.83,44.83 21.21,45.21 22.99,45.21 | D3.C 29.59,52.7 29.08,52.2 v27.81,52.2 | C5.2 27.94,53.09 27.81,52.96 v27.81,52.2 | C4.2 26.16,52.83 26.8,52.2 v27.81,52.2 | S1.2 8.81,9.73 10.16,8.38 v11.68,8.38 13.59,8.38 14.81,9.6 S1.1 | C21.2 v7.11,21.97 | J2.5 26.29,5.08 26.67,4.7 v26.92,4.7 27.18,4.7 27.56,5.08 J2.7 | J2.11 v30.1,4.7 | J3.13 45.72,59.05 46.1,58.67 v46.86,58.67 48.01,58.67 48.26,58.93 J3.14 | U1.74 52.11,42.33 52.6,42.82 v52.6,43.05 53.08,43.05 53.33,43.3 57.41,43.3 60.45,40.26 60.45,31.87 J4.10 | v15.11,58.8 15.24,58.93 J3.1 | U1.10 30.35,38.33 v30.35,38.35 | v34.42,45.59 33.5,44.68 U1.99 | U1.27 35.56,28.98 35.84,28.7 35.81,28.7 35.69,28.83 v35.69,29.21 | R3.2 38.1,49.96 v38.1,51.05 | D4.C 14.86,26.04 15.75,25.15 v21.34,25.15 | J4.12 78.36,28.66 J4.13 | J4.13 77.46,35.02 IC1.1 | J4.10 61.09,27.68 61.09,21.73 J4.11 | J4.13 73.87,29.56 73.32,29 67.9,29 67.31,29.59 | 66.72,29 | 66.72,29 66.87,29.15 66.87,29.56 J4.6
  Top 0.203: J4.10 63.15,29.46 63.61,29 66.72,29
  Top 0.305: C2.2 18.42,48.39 18.8,48.01 v19.43,48.01 19.81,48.01 20.45,48.64 C3.2 | U2.2 v23.24,51.82 | U2.7 v20.57,54.74
  pour Route2: 1.91,73.15 1.91,1.27 89.66,1.27 89.66,73.15
I2C1_SCL
  Top 0.203: U1.92 39.73,44.68 41.02,45.97 41.27,45.97 41.4,46.1 41.4,46.61 | R5.1 40.77,45.97 41.4,46.61 | 41.4,46.61 42.54,47.75 42.54,50.29 33.66,59.18 33.27,59.18 33.02,59.44 J3.8
I2C1_SDA
  Top 0.203: 38.86,51.5 34.2,46.84 U1.93 | 38.86,51.5 38.86,51.69 30.48,60.07 J3.7 | 38.86,51.5 38.86,47.24 40,46.1
LED-G
  Top 0.203: D2.A R2.1
LED-R
  Top 0.203: R1.1 D1.A
LED_G  (via drill 0.35)
  Top 0.203: U1.39 37.2,25.53 38.61,25.53 38.99,25.15 38.99,24.77 38.99,24.64 | 38.99,24.64 R2.2 | J3.10 38.1,58.8 v37.46,58.17 | v46.1,27.85 42.51,24.26 38.61,24.26 38.99,24.64
  Bottom 0.203: v37.46,58.17 37.46,30.86 37.72,30.61 42.93,30.61 44.45,29.08 44.45,28.32 44.92,27.85 v46.1,27.85
LED_R  (via drill 0.35)
  Top 0.203: U1.37 40.37,28.98 v41.5,27.85 38.79,25.14 35.7,25.14 35.81,25.02 37.34,25.02 37.72,24.64 R1.2 | J3.9 35.56,58.8 36.2,58.17 v36.45,58.17
  Bottom 0.203: v36.45,58.17 36.45,30.86 39.24,28.07 41.28,28.07 v41.5,27.85
MISO
  Top 0.203: J5.3 60.83,57.02 60.83,67.82 | 60.83,67.82 60.83,67.94 | V1.11 69.98,67.82 60.83,67.82
MOSI
  Top 0.203: R7.1 66.8,57.26 J5.4
N$1  (via drill 0.35)
  Top 0.203: U1.25 27.46,32.23 26.57,32.23 v26.54,32.26 | v17.91,27.3 19.62,25.6 23.82,25.6 24.13,25.91 16.96,25.91 D4.A
  Bottom 0.203: v26.54,32.26 20.32,26.04 17.91,26.04 v17.91,27.3
N$2
  Top 0.203: U1.33 37.43,28.98 37.43,28.49 37.57,28.35 37.87,28.35 38.07,28.55 38.07,28.85 38.03,28.9 38.03,29.13 37.82,29.34 37.52,29.34 37.42,29.23 37.32,29.34 37.02,29.34 36.72,29.03 36.72,28.42 36.57,28.27 36.57,27.98 36.78,27.77 36.69,27.68 35.68,27.68 28.54,20.54 28.54,23.84 28.07,23.37 28.07,19 31.06,16 USART3.2
N$3  (via drill 0.35)
  Top 0.203: v40.64,31.24 38.38,28.98 U1.34 | v44.7,25.4 44.7,20.14 40.56,16 USART3.1
  Bottom 0.203: v40.64,31.24 40.64,29.46 v44.7,25.4
N$4
  Top 0.203: U1.78 43.21,44.68 USART4.2
N$5
  Top 0.203: U1.69 44.55,39.34 USART1.2
N$6
  Top 0.203: USART4.1 41.2,45.57 U1.79
N$7
  Top 0.203: U1.70 46.46,40.33 USART1.1
N$9
  Top 0.203: V1.2 R7.2
N$10
  Top 0.203: V1.9 76.84,71.75 76.96,71.88 81.79,71.88 83.19,70.49 R10.2
N$11
  Top 0.203: U1.18 27.46,35.73 26.5,35.73 26.29,35.94 C1.2
N$13
  Top 0.203: R11.2 74.03,61.98 V1.5
N$14
  Top 0.203: R6.1 D3.A
N$17
  Top 0.203: R12.2 59.07,71.37 68.58,71.37 69.22,70.74 V1.12
NRST  (via drill 0.35)
  Top 0.203: S1.4 8.81,17.65 | 8.81,17.65 8.81,17.73 8.25,18.29 7.62,18.29 | 7.62,18.29 R9.2 | 7.62,18.29 7.11,18.8 C21.1 | S1.3 14.86,15.89 14.86,17.65 13.33,19.18 13.33,20.57 11.05,22.86 | 8.81,17.65 11.05,19.89 11.05,22.86 | 11.05,22.86 11.05,26.67 | 11.05,26.67 11.05,43.43 14.73,47.12 21.34,47.12 25.78,51.56 29.59,51.56 30.73,52.7 30.73,54.36 | 30.73,54.36 30.73,57.15 29.46,58.42 25.91,58.42 25.53,58.8 25.53,60.71 J3.5 | J2.12 30.1,14.1 23.75,20.45 17.27,20.45 11.05,26.67 | U1.14 27.46,37.73 27.06,37.73 v26.29,36.96 | v32.13,52.96 30.73,54.36
  Bottom 0.203: v26.29,36.96 25.65,37.59 25.65,46.48 v32.13,52.96
PC14-OSC32-IN
  Top 0.203: U1.8 27.46,40.73 26.71,40.73 25.97,41.47 | Y2.2 25.21,42.23 25.97,41.47 | 25.97,41.47 25.97,42.34 C8.1
PC15-OSC32-OUT  (via drill 0.35)
  Top 0.203: C9.1 19.96,43.16 19.56,43.56 v19.18,43.56 | v24.38,39.5 24.77,39.88 Y2.1 25.97,40.83 26.43,40.37 27.07,40.37 28.61,38.83 U1.9
  Bottom 0.203: v19.18,43.56 18.8,43.18 18.8,42.42 21.72,39.5 v24.38,39.5
SCK
  Top 0.203: R11.1 70.1,54.36 J5.5
SCK_LLS
  Top 0.203: J4.5 68.46,49.03 70.69,51.26 70.69,53.83 76.84,59.98 V1.6
SWCLK  (via drill 0.35)
  Top 0.203: U1.76 47.6,44.68 49.15,46.23 v49.66,46.23 | J2.6 26.29,9.14 26.54,8.89 28.45,8.89 28.83,8.51 J2.9 28.83,4.19 29.34,3.68 55.75,3.68 55.44,3.37 v55.44,8.18
  Bottom 0.203: v49.66,46.23 43.06,46.23 42.43,45.6 41.9,45.6 41.53,45.97 41.53,46.61 43.03,48.11 56.64,48.11 56.64,8.18 v55.44,8.18
SWDIO  (via drill 0.35)
  Top 0.203: J2.4 25.02,13.97 29.34,18.29 v29.34,19.05 | v52.32,41.27 44.61,41.27 U1.72
  Bottom 0.203: v29.34,19.05 34.54,13.84 40,13.84 48.01,21.84 48.01,36.96 v52.32,41.27
SWO  (via drill 0.35)
  Top 0.203: v42.16,46.23 40.62,44.68 U1.89 | J2.8 27.56,13.84 30.1,16.38 v30.1,18.16
  Bottom 0.203: v30.1,18.16 35.31,12.95 50.04,12.95 55.88,18.8 55.88,46.86 55.12,47.62 43.05,47.62 42.16,46.74 v42.16,46.23
USART_RX  (via drill 0.35)
  Top 0.203: U1.87 37.2,46.84 40,49.64 40,60.2 J3.11 40.51,60.96 40.51,62.36 41.91,63.75 53.47,63.75 54.23,62.99 v54.23,50.93 | J2.13 31.37,4.83 31.75,4.45 48.39,4.45 53.97,10.03 v55.37,10.03 | 54.36,49.02 v54.23,49.02
  Bottom 0.203: v54.23,50.93 v54.23,49.02 57.28,45.97 57.28,11.56 55.75,10.03 v55.37,10.03
USART_TX  (via drill 0.35)
  Top 0.203: U1.86 43.18,50.16 J3.12 43.18,62.23 43.81,62.87 52.83,62.87 53.09,62.61 v53.09,50.93 | J2.14 31.37,9.27 31.75,8.89 32.89,8.89 33.66,8.13 33.66,5.59 34.04,5.21 45.47,5.21 v49.4,9.14
  Bottom 0.203: v53.09,50.93 v53.09,49.02 53.09,12.83 v49.4,9.14
VDDA
  Top 0.203: U1.22 27.46,33.73 26.49,33.73 25.53,32.77 25.53,32.51 | 25.53,32.51 25.53,30.69 C18.A | R8.2 25.53,32.51 | C18.A 25.61,30.32 C17.1 | C18.A 24.73,29.73 FB1.1
VIN  (via drill 0.35)
  Top 0.203: IC1.3 87.12,40.06 v87.12,46.35 | v61.72,51.05 J5.2
  Route15 0.203: v87.12,46.35 66.42,46.35 v61.72,51.05
VREF_PLUS
  Top 0.203: U1.21 27.52,34.16 26.16,34.16 25.64,33.64 C19.1 24.11,33.64 23.83,33.35 R8.1 22.73,32.51 21.72,33.53 C20.A

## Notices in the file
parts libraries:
SparkFun-Connectors: Licensing: Creative Commons ShareAlike 4.0 International - https://creativecommons.org/licenses/by-sa/4.0
